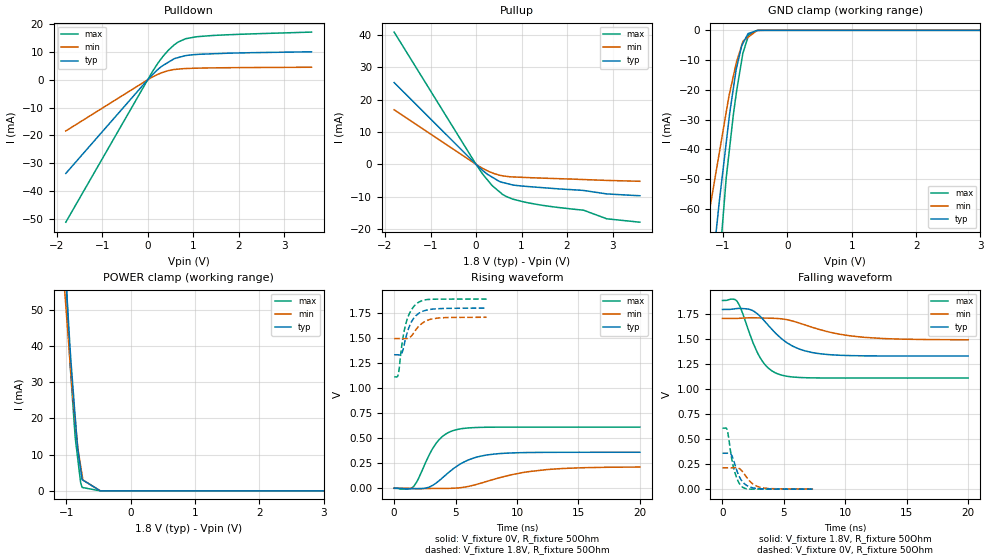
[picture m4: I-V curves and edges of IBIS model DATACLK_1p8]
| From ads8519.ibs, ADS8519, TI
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|   dataclk_1p8 Model
[Model]   DATACLK_1p8
Model_type   I/O
Polarity   Non-Inverting
Enable   Active-Low
Vinl = 0.6
Vinh = 0.945
Vmeas = 0.9
Vref = 0.9
Cref = 15pF
Rref = 50
|   typ   min   max
|   (nom PVT)   (Fast PVT)   (slow PVT)
| C_comp by Frequency method (F=29Mhz)
|Average
C_comp   1.0987e-11  1.002e-11   1.205e-11
|ON state : BUFFER OUTPUT TURNED HIGH
|C_comp   1.220e-11   1.118e-11   1.317e-11
|OFF state: BUFFER IN HIGH IMPEDANCE
|C_comp   9.952e-12   8.866e-12   1.094e-11
| C_comp by LC Tank method (L=1nH)
| Average
| Resonant frequency (Hz)   1.67e9   1.73e9   1.61e9
| C_comp   9.092e-12   8.472e-12   9.782e-12
| Where nom  PVT is Nominal Process,  1.8V,  32C
|   Fast PVT is Strong Process,   1.89V,  -40C
|   Slow PVT is Weak Process,   1.71V,  92C
[Model Spec]
Vinl   0.6   0.6   0.6
Vinh   0.9   0.855   0.945
[Voltage Range]   1.8   1.71   1.89
|Ambient Temperature   25   85   -40
|Junction Temperature
[Temperature Range]   32   92   -40
[Pullup Reference]   1.8   1.71   1.89
[Pulldown Reference]   0   0   0
[Power Clamp Reference]   1.8   1.71   1.89
[GND Clamp Reference]   0   0   0
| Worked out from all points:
|   slope of the pulldown table from 0 to 0.27 V, typ, clamps not added: 62.1 ohm
|   slope of the pullup table from 0 to 0.27 V, typ, clamps not added: 83.6 ohm
|   GND clamp passes 1 mA (typ) near -0.60 V on its own axis
|   falling waveform, V_fixture 1.8V, R_fixture 50Ohm: 20-80 % time 2.57ns typ, 4.05ns min, 1.61ns max; typ from 1.8 V to 1.33 V
|   rising waveform, V_fixture 0V, R_fixture 50Ohm: 20-80 % time 2.53ns typ, 4.39ns min, 1.62ns max; typ from 0 V to 0.36 V
|   rising waveform, V_fixture 1.8V, R_fixture 50Ohm: 20-80 % time 839ps typ, 990ps min, 732ps max; typ from 1.33 V to 1.8 V
|   falling waveform, V_fixture 0V, R_fixture 50Ohm: 20-80 % time 734ps typ, 915ps min, 600ps max; typ from 0.36 V to 0 V
[Pulldown]
|   Voltage   I(typ)   I(min)   I(max)
-1.8V     -33.72mA   -18.44mA   -51.27mA
107.7mV   1.898mA    1.028mA    3.036mA
332.6mV   5.099mA    2.665mA    8.353mA
451.7mV   6.282mA    3.26mA     10.59mA
574.6mV   7.501mA    3.675mA    12.46mA
667.2mV   7.982mA    3.83mA     13.56mA
835.4mV   8.687mA    4.034mA    14.78mA
1.089V    9.115mA    4.171mA    15.5mA
1.784V    9.568mA    4.338mA    16.21mA
3.6V      10.06mA    4.501mA    17.16mA
[GND Clamp]
|   Voltage   I(typ)   I(min)   I(max)
-1.8V     -221.7mA   -148.8mA   -315.6mA
-1.258V   -98.85mA   -66.66mA   -140.1mA
-1.217V   -90.37mA   -61.43mA   -126.9mA
-1.058V   -57.58mA   -41.21mA   -78.6mA
-952.6mV  -38.11mA   -27.73mA   -50.1mA
-894.6mV  -27.52mA   -20.77mA   -38.84mA
-837.3mV  -19.12mA   -15.17mA   -27.87mA
-797.4mV  -13.28mA   -11.27mA   -21.65mA
-693.6mV  -4.496mA   -3.903mA   -7.888mA
-612mV    -1.103mA   -2.341mA   -2.201mA
-444.6mV  -19.03uA   -20.98uA   -16.07uA
3.6V      0A         0A         0A
[Pullup]
|   Voltage   I(typ)   I(min)   I(max)
-1.8V     25.22mA    16.83mA    40.8mA
0V        0A         0A         0A
139.9mV   -1.811mA   -1.196mA   -2.9mA
332.6mV   -3.76mA    -2.487mA   -6.214mA
574.6mV   -5.558mA   -3.533mA   -9.177mA
801.4mV   -6.341mA   -3.882mA   -10.71mA
1.058V    -6.749mA   -4.037mA   -11.62mA
1.542V    -7.281mA   -4.293mA   -12.81mA
2.364V    -8.063mA   -4.693mA   -14.15mA
2.873V    -9.123mA   -4.96mA    -16.8mA
3.6V      -9.681mA   -5.228mA   -17.85mA
[POWER Clamp]
|   Voltage   I(typ)   I(min)   I(max)
-1.8V     356.9mA    291.2mA    437.2mA
-1.019V   62.09mA    53.29mA    63.54mA
-948.8mV  41.08mA    37mA       36.81mA
-913.1mV  31.99mA    28.77mA    27.45mA
-863.7mV  20.48mA    19.56mA    14.85mA
-835.2mV  13.83mA    14.24mA    10.63mA
-820.8mV  11.24mA    11.56mA    8.504mA
-778.7mV  5.968mA    6.879mA    2.282mA
-756mV    3.127mA    4.36mA     963.5uA
-743.9mV  2.993mA    3.011mA    922.4uA
-470.3mV  154.4nA    1.044uA    3.966nA
3.6V      0A         0A         0A
[Ramp]
R_load = 50
|   typ   min   max
dV/dt_r   0.215874/2.51861e-09   0.12739/4.35061e-09   0.366667/1.61458e-09
dV/dt_f   0.279982/2.56413e-09   0.128284/4.04584e-09   0.466189/1.61005e-09
[Falling Waveform]
V_fixture = 1.8V
V_fixture_min = 1.71V
V_fixture_max = 1.89V
R_fixture = 50Ohm
|   Time   V(typ)   V(min)   V(max)
0s        1.8V       1.71V      1.89V
1.175ns   1.809V     1.71V      1.883V
2.25ns    1.799V     1.717V     1.545V
3.05ns    1.732V     1.715V     1.32V
3.8ns     1.631V     1.712V     1.205V
4.7ns     1.519V     1.707V     1.146V
6.15ns    1.409V     1.668V     1.119V
8ns       1.355V     1.595V     1.114V
11.53ns   1.335V     1.521V     1.113V
20ns      1.333V     1.496V     1.113V
[Rising Waveform]
V_fixture = 0V
V_fixture_min = 0V
V_fixture_max = 0V
R_fixture = 50Ohm
|   Time   V(typ)   V(min)   V(max)
0s        1.676nV    2.081nV    1.371nV
1.55ns    -4.1mV     -2.526mV   14.7mV
2.625ns   3.638mV    -2.821mV   274.3mV
3.45ns    55.35mV    -1.464mV   454.6mV
4.2ns     133mV      -1.102mV   541.6mV
5.075ns   218.2mV    2.036mV    585.6mV
6.55ns    305.2mV    33.49mV    606.5mV
8.575ns   346.5mV    105.4mV    610.7mV
12.47ns   358.9mV    187.2mV    611.1mV
20ns      359.8mV    212.3mV    611.1mV
[Rising Waveform]
V_fixture = 1.8V
V_fixture_min = 1.71V
V_fixture_max = 1.89V
R_fixture = 50Ohm
|   Time   V(typ)   V(min)   V(max)
0s        1.333V     1.495V     1.113V
275ps     1.333V     1.496V     1.116V
350ps     1.333V     1.496V     1.144V
700ps     1.375V     1.495V     1.49V
1.025ns   1.538V     1.496V     1.674V
1.375ns   1.654V     1.517V     1.775V
1.8ns     1.727V     1.589V     1.841V
2.45ns    1.773V     1.662V     1.88V
3.225ns   1.791V     1.695V     1.889V
7.525ns   1.8V       1.708V     1.89V
[Falling Waveform]
V_fixture = 0V
V_fixture_min = 0V
V_fixture_max = 0V
R_fixture = 50Ohm
|   Time   V(typ)   V(min)   V(max)
0s        359.8mV    213.6mV    611.1mV
375ps     359.9mV    213.5mV    594.7mV
475ps     361.1mV    213.4mV    536.8mV
675ps     352mV      213.5mV    363.3mV
950ps     273.1mV    214.4mV    192.9mV
1.3ns     144.6mV    210.1mV    73.29mV
1.65ns    71.5mV     172.6mV    18.63mV
2.35ns    17.22mV    64.39mV    -87.05uV
3.05ns    4.575mV    19.24mV    729.7uV
7.375ns   312uV      1.327mV    10.17uV
